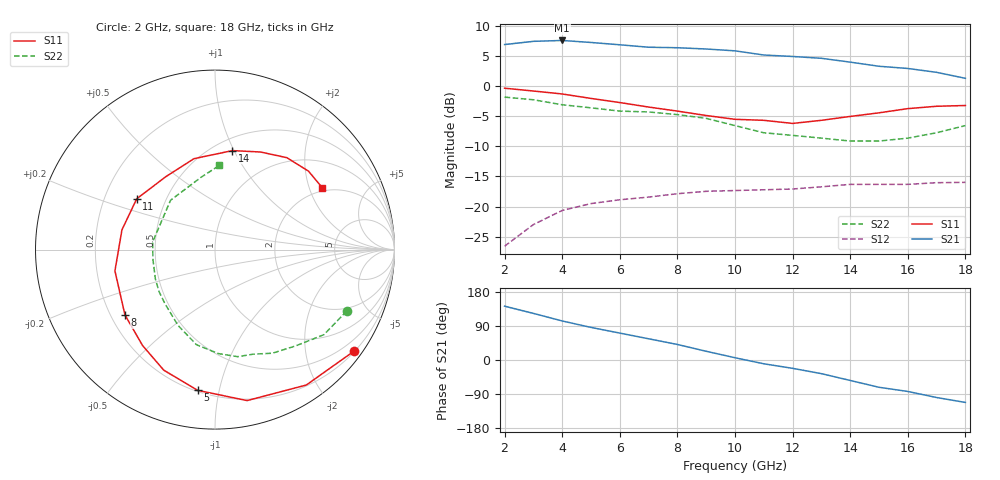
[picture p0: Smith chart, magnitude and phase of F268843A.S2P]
!ATF-26884
!S-PARAMETERS at Vds=3V  Id=10mA.  LAST UPDATED 07-22-92
# ghz s ma r 50
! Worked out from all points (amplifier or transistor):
!   17 points, 2 GHz to 18 GHz, reference 50 ohm
!   highest |S21| = 7.6 dB at 4 GHz (marker M1)
!   |S21| within 3 dB of that: start of sweep to 13.06 GHz
!   unconditionally stable (mu >= 1): 9.467 GHz to end of sweep
!   at 4 GHz: K = 0.44, MSG = 14.1 dB, |S12| = -20.6 dB
!   at 10 GHz: K = 1.07, MAG = 10.0 dB, |S12| = -17.3 dB
!   at 18 GHz: K = 1.03, MAG = 7.5 dB, |S12| = -16.0 dB
!   S11 on the Smith chart (normalised r, x): 2 GHz: 0.21, -3.06; 5 GHz: 0.21, -0.86; 8 GHz: 0.26, -0.31; 11 GHz: 0.34, +0.26; 14 GHz: 0.61, +0.99; 18 GHz: 1.86, +2.46
2  0.96 -36.0  2.21 142.0  0.047 64.0  0.81 -25.0
3  0.91 -56.0  2.35 123.0  0.071 50.0  0.77 -38.0
4  0.86 -78.0  2.39 103.0  0.093 36.0  0.7 -50.0
5  0.79 -97.0  2.3 86.0  0.106 25.0  0.66 -61.0
6  0.73 -113.0  2.2 71.0  0.114 16.0  0.62 -70.0
7  0.67 -127.0  2.1 56.0  0.12 9.0  0.61 -78.0
8  0.62 -144.0  2.08 41.0  0.128 1.0  0.58 -88.0
9  0.57 -168.0  2.03 23.0  0.134 -8.0  0.54 -101.0
10  0.53 168.0  1.96 6.0  0.136 -16.0  0.47 -116.0
11  0.52 147.0  1.81 -10.0  0.138 -22.0  0.41 -133.0
12  0.49 124.0  1.76 -22.0  0.14 -26.0  0.39 -143.0
13  0.52 103.0  1.7 -36.0  0.146 -31.0  0.37 -154.0
14  0.56 80.0  1.58 -54.0  0.153 -37.0  0.35 -171.0
15  0.6 65.0  1.46 -72.0  0.153 -42.0  0.35 173.0
16  0.65 52.0  1.4 -83.0  0.153 -48.0  0.37 132.0
17  0.68 40.0  1.3 -99.0  0.158 -56.0  0.41 101.0
18  0.69 30.0  1.16 -112.0  0.159 -72.0  0.47 87.0
